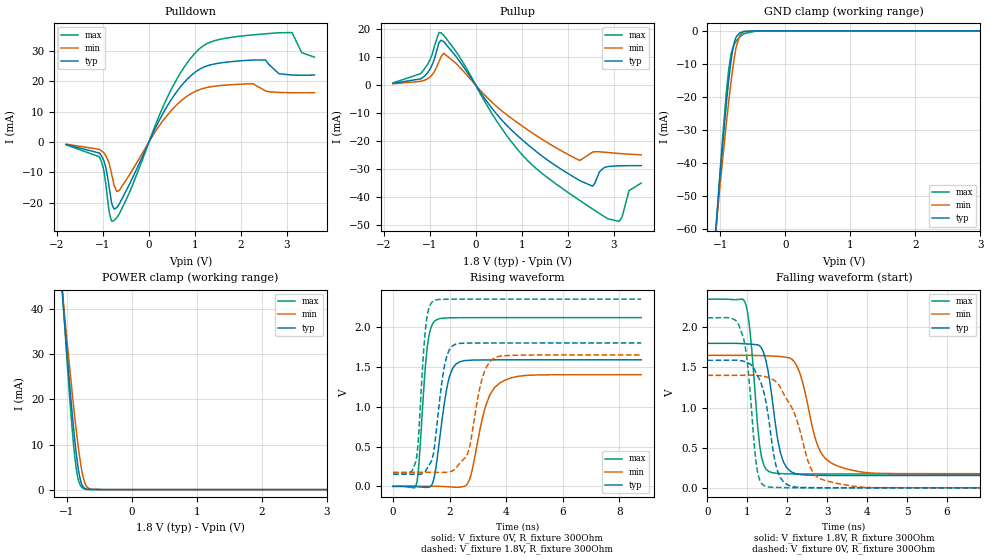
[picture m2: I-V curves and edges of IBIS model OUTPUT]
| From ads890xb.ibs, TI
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|   OUTPUT_300M
[Model]   OUTPUT
Model_type   3-state
Polarity   Non-Inverting
Vmeas = 0.9
Vref = 0
Cref = 2pF
Rref = 300
|   typ   min   max
C_comp   1.41788E-12  1.32935E-12  1.45761E-12
|Where Nom  PVT is Nominal Process,  1.8V,  25C
|   Fast PVT is Strong Process,  2.35V, 0C
|   Slow PVT is Weak Process,   1.65V, 60C
[Voltage Range]   1.8   1.65   2.35
[Temperature Range]   25   60   0
[Pullup Reference]   1.8   1.65   2.35
[Pulldown Reference]   0   0   0
[Power Clamp Reference]   1.8   1.65   2.35
[GND Clamp Reference]   0   0   0
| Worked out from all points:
|   slope of the pulldown table from 0 to 0.27 V, typ, clamps not added: 32 ohm
|   slope of the pullup table from 0 to 0.27 V, typ, clamps not added: 41.9 ohm
|   GND clamp passes 1 mA (typ) near -0.72 V on its own axis
|   POWER clamp passes 1 mA (typ) near -0.76 V on its own axis
|   falling waveform, V_fixture 1.8V, R_fixture 300Ohm: 20-80 % time 296ps typ, 449ps min, 217ps max; typ from 1.8 V to 0.153 V
|   rising waveform, V_fixture 0V, R_fixture 300Ohm: 20-80 % time 377ps typ, 551ps min, 251ps max; typ from 0 V to 1.59 V
|   rising waveform, V_fixture 1.8V, R_fixture 300Ohm: 20-80 % time 342ps typ, 458ps min, 234ps max; typ from 0.153 V to 1.8 V
|   falling waveform, V_fixture 0V, R_fixture 300Ohm: 20-80 % time 334ps typ, 592ps min, 229ps max; typ from 1.59 V to 0 V
[Pulldown]
|   Voltage   I(typ)   I(min)   I(max)
-1.8V     -839.7uA   -686.5uA   -928uA
-1.082V   -3.627mA   -2.418mA   -4.847mA
-941.4mV  -8.209mA   -4.413mA   -13.58mA
-860.4mV  -15.45mA   -7.396mA   -23.46mA
-801mV    -20.72mA   -11.31mA   -26.13mA
-644.4mV  -20.38mA   -15.93mA   -23.65mA
462.6mV   13.45mA    10.01mA    16.66mA
1.116V    24.11mA    17.36mA    30.95mA
2.536V    27.03mA    16.82mA    35.67mA
3.109V    22.07mA    16.23mA    36.08mA
3.325V    22.03mA    16.23mA    29.46mA
3.6V      22.06mA    16.25mA    27.99mA
[GND Clamp]
|   Voltage   I(typ)   I(min)   I(max)
-1.8V     -251.5mA   -220.6mA   -289.3mA
-1.152V   -79.8mA    -77.28mA   -85.14mA
-1.017V   -46.37mA   -49.15mA   -45.84mA
-968.4mV  -35mA      -39.43mA   -32.79mA
-909mV    -22.05mA   -28.05mA   -18.67mA
-849.6mV  -11.03mA   -17.55mA   -8.586mA
-784.8mV  -3.385mA   -7.983mA   -3.944mA
-752.4mV  -1.685mA   -4.472mA   -2.94mA
-703.8mV  -638.5uA   -1.379mA   -1.873mA
-639mV    -185.2uA   -197.8uA   -870.6uA
-439.2mV  -1.292uA   -461.3nA   -12.53uA
3.6V      0A         0A         0A
[Pullup]
|   Voltage   I(typ)   I(min)   I(max)
-1.8V     692.6uA    518.6uA    851.1uA
-1.12V    3.192mA    1.778mA    5.775mA
-757.8mV  16.11mA    10.2mA     18.79mA
-439.2mV  10.49mA    7.981mA    12.29mA
694.8mV   -14.69mA   -10.83mA   -18.47mA
1.597V    -27.18mA   -20.91mA   -33.5mA
2.266V    -34.15mA   -26.93mA   -41.28mA
2.536V    -36.09mA   -23.96mA   -44.24mA
2.795V    -29.46mA   -23.95mA   -47.01mA
3.114V    -28.82mA   -24.42mA   -48.68mA
3.335V    -28.79mA   -24.68mA   -37.67mA
3.6V      -28.77mA   -24.89mA   -35.03mA
[POWER Clamp]
|   Voltage   I(typ)   I(min)   I(max)
-1.8V     191.1mA    166.2mA    221.9mA
-1.082V   45.76mA    45.99mA    47.3mA
-1.017V   33.82mA    36.05mA    32.98mA
-936mV    19.85mA    24.11mA    16.67mA
-876.6mV  10.84mA    15.95mA    7.177mA
-849.6mV  7.377mA    12.51mA    4.155mA
-822.6mV  4.518mA    9.336mA    2.159mA
-790.2mV  2.102mA    5.99mA     901.6uA
-752.4mV  673uA      2.984mA    306uA
-703.8mV  121.7uA    857.8uA    67.21uA
-639mV    11.12uA    105.9uA    7.757uA
3.6V      0A         0A         0A
[Ramp]
R_load = 300
|   typ   min   max
dV/dt_r   0.953007/3.76552e-10   0.840788/5.50756e-10   1.27073/2.51028e-10
dV/dt_f   0.988106/2.95941e-10   0.884269/4.49376e-10   1.30677/2.17498e-10
[Falling Waveform]
V_fixture = 1.8V
V_fixture_min = 1.65V
V_fixture_max = 2.35V
R_fixture = 300Ohm
C_fixture = 0F
|   Time   V(typ)   V(min)   V(max)
0s        1.8V       1.65V      2.35V
945.4ps   1.794V     1.65V      2.305V
1.074ns   1.79V      1.65V      1.911V
1.306ns   1.771V     1.647V     535.5mV
1.547ns   1.367V     1.643V     201.7mV
1.824ns   445.3mV    1.635V     177.7mV
2.211ns   175.4mV    1.541V     173.5mV
2.753ns   156mV      536.4mV    172.7mV
3.266ns   154mV      271mV      172.3mV
8.773ns   153.1mV    176.2mV    172mV
[Rising Waveform]
V_fixture = 0V
V_fixture_min = 0V
V_fixture_max = 0V
R_fixture = 300Ohm
C_fixture = 0F
|   Time   V(typ)   V(min)   V(max)
0s        14.36uV    15.37uV    8.204uV
829.9ps   -2.229mV   25.84uV    33.75mV
1.217ns   -13.07mV   30.71uV    1.765V
1.478ns   154.6mV    34.01uV    2.076V
1.907ns   1.244V     -4.564mV   2.114V
2.345ns   1.562V     -10.27mV   2.117V
2.693ns   1.582V     76.42mV    2.117V
3.266ns   1.587V     1.001V     2.118V
3.795ns   1.588V     1.302V     2.118V
8.773ns   1.588V     1.401V     2.118V
[Rising Waveform]
V_fixture = 1.8V
V_fixture_min = 1.65V
V_fixture_max = 2.35V
R_fixture = 300Ohm
C_fixture = 0F
|   Time   V(typ)   V(min)   V(max)
0s        153.1mV    176.2mV    172mV
804.3ps   151.5mV    176.2mV    313.5mV
1.15ns    192.4mV    176.1mV    1.987V
1.418ns   396.1mV    175.7mV    2.326V
1.824ns   1.523V     175.7mV    2.348V
2.096ns   1.763V     194.2mV    2.349V
2.623ns   1.798V     399.1mV    2.349V
3.163ns   1.799V     1.371V     2.35V
3.594ns   1.799V     1.615V     2.35V
8.773ns   1.8V       1.65V      2.35V
[Falling Waveform]
|Gnd
V_fixture = 0V
V_fixture_min = 0V
V_fixture_max = 0V
R_fixture = 300Ohm
C_fixture = 0F
|   Time   V(typ)   V(min)   V(max)
0s        1.588V     1.401V     2.118V
883.9ps   1.579V     1.403V     1.893V
1.008ns   1.558V     1.404V     1.525V
1.217ns   1.435V     1.401V     317.6mV
1.418ns   1.178V     1.388V     27.12mV
1.759ns   203.5mV    1.301V     4.995mV
2.096ns   20.41mV    1.014V     1.398mV
2.572ns   3.273mV    262.2mV    1.1mV
2.934ns   1.181mV    94.18mV    1.036mV
8.773ns   12.88uV    15.33uV    8.221uV
